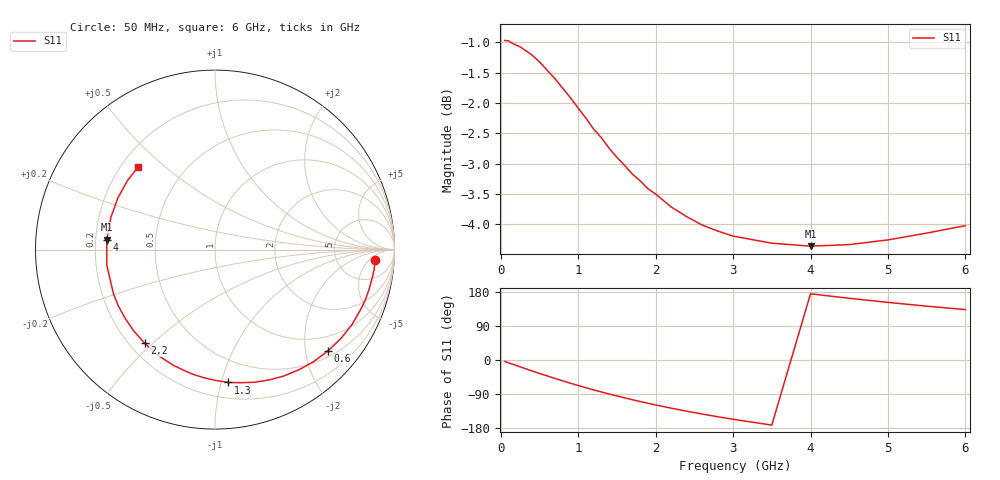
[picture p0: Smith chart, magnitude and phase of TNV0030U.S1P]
! SIEMENS Discrete & RF Semiconductors
! BAS70-07W
! Si Schottky Diode in SOT343
! IF = 0.03 mA
! S-Parameters:  February  1997
# GHz  S  MA  R  50
!  f  S11
! GHz  MAG  ANG
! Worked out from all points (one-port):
!   34 points, 50 MHz to 6 GHz, reference 50 ohm
!   lowest |S11| = -4.4 dB at 4 GHz (marker M1), VSWR 4.07, Z = 12.3 + j2.17 ohm
!   |S11| at or under -10 dB: nowhere
!   S11 on the Smith chart (normalised r, x): 50 MHz: 13, -8; 600 MHz: 0.62, -2.47; 1.3 GHz: 0.32, -1.05; 2.2 GHz: 0.26, -0.47; 4 GHz: 0.25, +0.04; 6 GHz: 0.27, +0.41
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0.05  0.8942 -3.7
0.15  0.8893 -10.9
0.3  0.8791 -21.5
0.4  0.8703 -28.5
0.5  0.8586 -35.3
0.6  0.8451 -42.0
0.7  0.8318 -48.6
0.8  0.8168 -55.0
0.9  0.8023 -61.3
1  0.7866 -67.3
1.1  0.7718 -73.2
1.3  0.7437 -84.4
1.5  0.7166 -94.9
1.6  0.7057 -99.9
1.8  0.6855 -109.6
1.9  0.6753 -114.1
2  0.6684 -118.6
2.2  0.6523 -127.0
2.4  0.6405 -135.0
2.6  0.6303 -142.6
2.8  0.6233 -149.7
3  0.6172 -156.4
3.5  0.609 -171.8
4  0.6056 174.7
4.5  0.6074 162.8
5  0.6128 152.0
5.5  0.6208 142.1
6  0.6296 133.0
